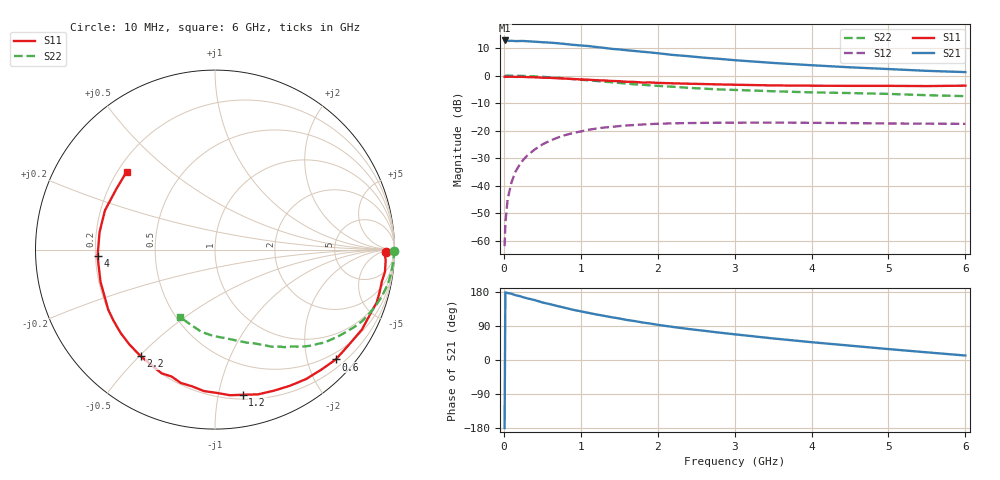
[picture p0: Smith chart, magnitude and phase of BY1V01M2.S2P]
! SIEMENS Small Signal Semiconductors
! BFY420
! Si NPN RF SIEGET Grounded Emitter Transistor in MICRO-X
! VCE = 1 V  IC = 1.2 mA
! Common Emitter S-Parameters:  October  1996
# GHz  S  MA  R  50
!  f  S11  S21  S12  S22
! GHz  MAG  ANG  MAG  ANG  MAG  ANG  MAG  ANG
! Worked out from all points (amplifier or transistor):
!   36 points, 10 MHz to 6 GHz, reference 50 ohm
!   highest |S21| = 12.8 dB at 10 MHz (marker M1)
!   |S21| within 3 dB of that: start of sweep to 1.386 GHz
!   unconditionally stable (mu >= 1): 4.413 GHz to end of sweep
!   at 250 MHz: K = 0.03, MSG = 21.6 dB, |S12| = -30.7 dB
!   at 1.4 GHz: K = 0.25, MSG = 14.2 dB, |S12| = -18.6 dB
!   at 6 GHz: K = 1.33, MAG = 6.0 dB, |S12| = -17.5 dB
!   S11 on the Smith chart (normalised r, x): 10 MHz: 39, -10; 600 MHz: 0.36, -2.54; 1.2 GHz: 0.24, -1.18; 2.2 GHz: 0.20, -0.50; 4 GHz: 0.21, -0.03; 6 GHz: 0.24, +0.36
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0.01  0.9535 -0.7  4.342 -179.4  0.0008 103.0  0.9984 -0.4
0.02  0.9474 -1.6  4.311 178.6  0.0021 90.3  0.9899 -0.7
0.05  0.9527 -3.7  4.251 176.7  0.0058 89.3  0.9969 -1.9
0.1  0.9551 -7.4  4.278 174.8  0.0116 85.2  0.9945 -3.9
0.15  0.9467 -10.7  4.23 171.0  0.0179 81.9  0.9916 -6.0
0.25  0.9479 -18.2  4.251 165.7  0.0292 78.7  0.9852 -9.8
0.4  0.9319 -28.5  4.121 158.2  0.0454 72.0  0.9664 -15.4
0.5  0.915 -35.6  4.034 151.9  0.0561 68.1  0.9495 -19.1
0.6  0.9097 -42.3  3.966 147.3  0.0658 63.7  0.9307 -22.6
0.8  0.8814 -55.1  3.742 137.4  0.0833 55.9  0.8877 -29.1
0.9  0.8652 -61.4  3.616 132.5  0.0906 52.4  0.8638 -32.0
1.1  0.8413 -73.5  3.437 124.4  0.1037 45.5  0.8194 -37.7
1.2  0.8234 -79.2  3.301 120.3  0.1091 42.5  0.7982 -40.5
1.6  0.7722 -99.7  2.88 105.6  0.1244 31.7  0.715 -49.2
2  0.7376 -117.6  2.547 92.8  0.1334 23.2  0.6502 -56.2
2.2  0.7236 -125.0  2.37 87.2  0.1359 19.5  0.6274 -59.6
2.8  0.6906 -144.9  2.013 72.3  0.1393 11.2  0.5608 -68.2
3.5  0.6626 -164.3  1.697 56.9  0.1404 4.3  0.5197 -76.9
4  0.6555 -176.8  1.542 47.0  0.1388 0.5  0.4959 -83.7
4.5  0.6504 171.4  1.413 37.9  0.1372 -2.8  0.4818 -90.8
5.5  0.6449 148.9  1.219 20.2  0.134 -5.9  0.4403 -107.7
6  0.6565 138.6  1.156 11.8  0.1331 -6.3  0.4232 -117.4
